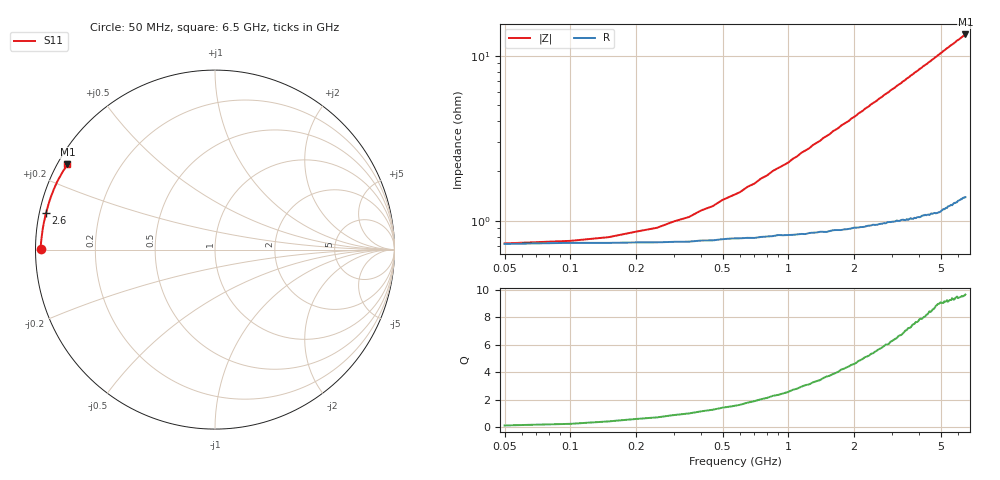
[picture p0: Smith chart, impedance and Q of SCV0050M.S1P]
! Infineon Technologies  Discrete & RF Semiconductors
! BAR63-02L
! Si PIN Diode in TSLP-2
! IF = 50 mA
! S-Parameters:  March  2002
# GHz  S  MA  R  50
!  f  S11
! GHz  MAG  ANG
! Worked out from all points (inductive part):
!   130 points, 50 MHz to 6.5 GHz, reference 50 ohm
!   read as one part to ground: L = 332 pH near 1.2 GHz
!   highest Q = 9.64 at 6.5 GHz (marker M1), where L = 328 pH
!   S11 on the Smith chart (normalised r, x): 50 MHz: 0.01, +0.00; 2.6 GHz: 0.02, +0.11; 6.5 GHz: 0.03, +0.27
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0.05  0.9715 179.8
0.5  0.9696 177.5
0.6  0.9692 177.1
0.9  0.9678 175.6
1  0.9678 175.2
1.15  0.9674 174.4
1.6  0.9658 172.3
1.7  0.9657 171.9
1.75  0.9657 171.6
1.9  0.9652 171.0
2.25  0.9642 169.3
2.5  0.9634 168.2
2.6  0.9631 167.7
3.1  0.9618 165.5
3.15  0.9613 165.2
3.3  0.9611 164.6
3.8  0.9602 162.2
4.1  0.9593 160.9
4.15  0.959 160.6
4.35  0.9587 159.8
4.9  0.9577 157.2
5.3  0.9554 155.3
5.7  0.9534 153.6
5.9  0.9524 152.6
6.15  0.9509 151.6
6.35  0.9498 150.6
6.4  0.9498 150.5
6.5  0.9495 150.0
